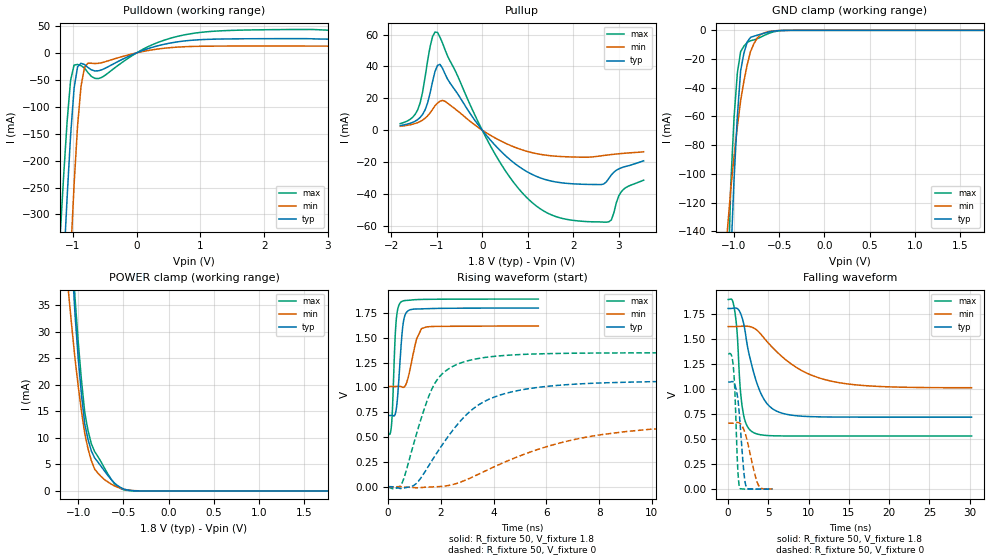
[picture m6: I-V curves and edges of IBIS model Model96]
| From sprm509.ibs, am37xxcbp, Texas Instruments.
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| Model based on original model for BQ18OMAPSMART1HYFBPBNOPM_SSBHV
|   Sub model PM_VS00L11_PUPD0_1P8
[model]   Model96
|[Input Load]   PI
|[Output Drive] SC00LB11
|Voltage   1.8V
|Mode   I/O
Model_type   I/O
Polarity   Non-Inverting
Enable   Active-Low
Vinl =  0.63
Vinh =  1.17
Cref =  15pF
Rref =  100.0000M
Vref =  0V
Vmeas =  0.9
C_comp   1.410688p   1.256095p   1.577871p
[Model Spec]
Vinl   0.63   0.567   0.6615
Vinh   1.17   1.053   1.2285
[Temperature Range]   25   125   -40
[Voltage Range]   1.8   1.62   1.89
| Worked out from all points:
|   slope of the pulldown table from 0 to 0.27 V, typ, clamps not added: 24.3 ohm
|   slope of the pullup table from 0 to 0.27 V, typ, clamps not added: 29.7 ohm
|   GND clamp passes 1 mA (typ) near -0.60 V on its own axis
|   POWER clamp passes 1 mA (typ) near -0.56 V on its own axis
|   rising waveform, R_fixture 50, V_fixture 1.8: 20-80 % time 176ps typ, 306ps min, 123ps max; typ from 0.718 V to 1.8 V
|   rising waveform, R_fixture 50, V_fixture 0: 20-80 % time 2.08ns typ, 4.62ns min, 1.07ns max; typ from 0 V to 1.07 V
|   falling waveform, R_fixture 50, V_fixture 1.8: 20-80 % time 2.1ns typ, 5.91ns min, 728ps max; typ from 1.8 V to 0.718 V
|   falling waveform, R_fixture 50, V_fixture 0: 20-80 % time 637ps typ, 1.14ns min, 381ps max; typ from 1.07 V to 0 V
[POWER_clamp]
-1.8V     362.5mA    191.4mA    412.8mA
-1.109V   56.69mA    37.71mA    60.38mA
-1.073V   44.6mA     31.22mA    47.8mA
-1.036V   33.44mA    25.04mA    36.59mA
-1V       24.98mA    19.72mA    28.06mA
-963.6mV  18.03mA    14.96mA    20.78mA
-927.3mV  12.59mA    10.77mA    14.74mA
-890.9mV  9.653mA    7.899mA    11.31mA
-818.2mV  6.214mA    4.114mA    7.414mA
-636.4mV  2.183mA    1.307mA    2.238mA
-418.2mV  83.85uA    105.2uA    35.14uA
1.764V    -1.228nA   -79.11nA   -1.453nA
[Pulldown]
-1.8V     -1.718A    -2.61A     -1.406A
-1.2V     -527.4mA   -844.5mA   -339.9mA
-1.145V   -396mA     -683.1mA   -229.1mA
-1.091V   -269mA     -526.7mA   -127.5mA
-1.036V   -153.6mA   -378.9mA   -51.17mA
-981.8mV  -66.34mA   -245.6mA   -22.67mA
-927.3mV  -26mA      -136.2mA   -21.54mA
-872.7mV  -19.34mA   -61.98mA   -23.69mA
-763.6mV  -27.2mA    -19.05mA   -36.72mA
-545.5mV  -31.39mA   -18.17mA   -45.46mA
872.7mV   23.46mA    11.88mA    35.92mA
3.545V    25.34mA    12.51mA    41.58mA
[Pullup]
-1.8V     2.903mA    2.423mA    4.112mA
-1.418V   6.595mA    4.711mA    12.64mA
-1.255V   12.69mA    7.42mA     33.23mA
-1.091V   30.4mA     13mA       58.69mA
-981.8mV  40.63mA    17.02mA    61.3mA
-818.2mV  35.38mA    18.12mA    50.59mA
272.7mV   -9.18mA    -4.728mA   -14.55mA
1.255V    -29.75mA   -15.09mA   -48.97mA
2.564V    -34.17mA   -16.31mA   -57.57mA
2.782V    -30.25mA   -15.5mA    -57.48mA
3.055V    -23.63mA   -14.68mA   -38.61mA
3.545V    -19.25mA   -13.56mA   -31.41mA
[GND_clamp]
-1.8V     -2.82A     -1.192A    -3.165A
-1.073V   -235.7mA   -138.4mA   -192.1mA
-1.036V   -159.5mA   -110.8mA   -107.5mA
-1V       -103.8mA   -87.85mA   -60.67mA
-963.6mV  -60mA      -67.28mA   -29.8mA
-927.3mV  -28.21mA   -49.08mA   -14.9mA
-890.9mV  -15.9mA    -35.48mA   -10.99mA
-854.5mV  -8.138mA   -24.07mA   -8.449mA
-818.2mV  -4.924mA   -14.85mA   -7.266mA
-709.1mV  -2.784mA   -3.064mA   -4.883mA
-563.6mV  -570.2uA   -404.5uA   -1.092mA
1.764V    -11.02pA   583.5nA    3.035nA
[Ramp]
dV/dt_f  0.6521835/2.0988n   0.3687351/5.954484n   0.8185908/0.7282378n
dV/dt_r  0.6518802/2.082618n   0.4008743/4.667954n   0.8245416/1.072475n
R_load = 50
[Rising Waveform]
R_fixture = 50
V_fixture = 1.8
V_fixture_min = 1.62
V_fixture_max = 1.89
0s        717.6mV    1.009V     531.8mV
144ps     719.8mV    1.009V     668.7mV
288ps     747.8mV    1.009V     1.601V
351ps     873.9mV    1.01V      1.767V
477ps     1.357V     1.01V      1.857V
558ps     1.616V     1.001V     1.87V
666ps     1.742V     1.024V     1.876V
1.08ns    1.79V      1.487V     1.884V
1.269ns   1.791V     1.593V     1.886V
5.697ns   1.799V     1.618V     1.89V
[Rising Waveform]
R_fixture = 50
V_fixture = 0
V_fixture_min = 0
V_fixture_max = 0
0s        -327.4uV   112.6uV    -3.55mV
540ps     -16.78mV   -593.3uV   42.4mV
1.08ns    35.02mV    -10.48mV   533.7mV
1.548ns   214.1mV    -2.993mV   914.3mV
1.854ns   342mV      361.7uV    1.075V
2.466ns   572.7mV    23.03mV    1.214V
3.51ns    837.3mV    136.7mV    1.295V
6.516ns   1.023V     440.9mV    1.343V
9.945ns   1.058V     578.6mV    1.348V
30.37ns   1.068V     655.8mV    1.349V
[Falling Waveform]
R_fixture = 50
V_fixture = 1.8
V_fixture_min = 1.62
V_fixture_max = 1.89
0s        1.8V       1.62V      1.89V
891ps     1.805V     1.62V      1.734V
1.179ns   1.797V     1.621V     1.482V
1.476ns   1.763V     1.622V     1.028V
1.89ns    1.662V     1.624V     749.2mV
3.087ns   1.187V     1.609V     566.7mV
4.797ns   854.9mV    1.474V     534.9mV
7.308ns   745.3mV    1.28V      530.1mV
14.57ns   718.1mV    1.051V     529.8mV
30.24ns   717.6mV    1.011V     529.8mV
[Falling Waveform]
R_fixture = 50
V_fixture = 0
V_fixture_min = 0
V_fixture_max = 0
0s        1.068V     657.3mV    1.349V
432ps     1.072V     657.3mV    1.328V
666ps     1.064V     657.6mV    1.199V
855ps     1.034V     660.1mV    937.4mV
1.179ns   911mV      664.9mV    224.2mV
1.44ns    696mV      657.2mV    11.34mV
1.962ns   160.4mV    590.3mV    975uV
2.259ns   19.75mV    516.4mV    400.1uV
3.717ns   452.2uV    47.07mV    47.77uV
5.499ns   134.2uV    1.637mV    9.236uV
